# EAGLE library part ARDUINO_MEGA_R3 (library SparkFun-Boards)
Arduino Mega R3 ATmega2560 R3 compatible footprint. SparkFun Products: Arduino Mega 2560 R3
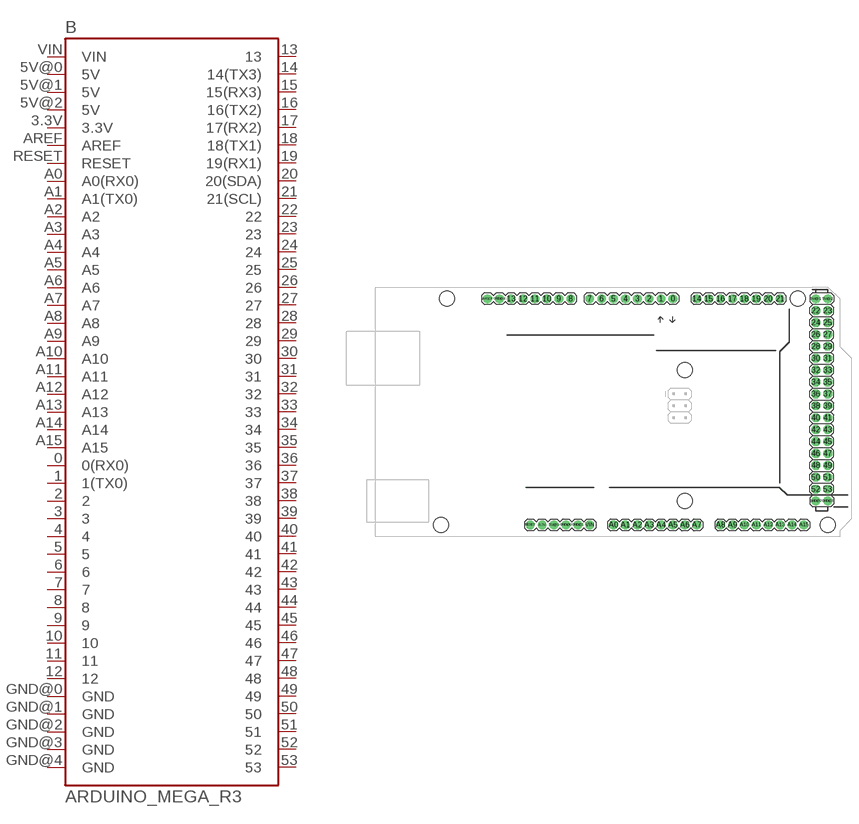
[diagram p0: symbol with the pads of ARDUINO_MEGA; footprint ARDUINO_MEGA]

Designator prefix B

## ARDUINO_MEGA_R3FULL  [ARDUINO_MEGA]
0  0(RX0)
1  1(TX0)
2  2
3  3
3.3V  3.3V
4  4
5  5
5V@0  5V
5V@1  5V
5V@2  5V
6  6
7  7
8  8
9  9
10  10
11  11
12  12
13  13
14  14(TX3)
15  15(RX3)
16  16(TX2)
17  17(RX2)
18  18(TX1)
19  19(RX1)
20  20(SDA)
21  21(SCL)
22  22
23  23
24  24
25  25
26  26
27  27
28  28
29  29
30  30
31  31
32  32
33  33
34  34
35  35
36  36
37  37
38  38
39  39
40  40
41  41
42  42
43  43
44  44
45  45
46  46
47  47
48  48
49  49
50  50
51  51
52  52
53  53
A0  A0(RX0)
A1  A1(TX0)
A2  A2
A3  A3
A4  A4
A5  A5
A6  A6
A7  A7
A8  A8
A9  A9
A10  A10
A11  A11
A12  A12
A13  A13
A14  A14
A15  A15
AREF  AREF
GND@0  GND
GND@1  GND
GND@2  GND
GND@3  GND
GND@4  GND
RESET  RESET
VIN  VIN

## Footprint ARDUINO_MEGA (pad centres in mm)
Arduino MEGA R3 footprint Specifications: Pin count:82 Area:4x2.15 in Example device(s): Arduino Mega R3
drill 1.016 pad 1.88: 0 13.97,24.13; 1 11.43,24.13; 2 8.89,24.13; 3 6.35,24.13; 3.3V -13.97,-24.13; 4 3.81,24.13; 5 1.27,24.13; 5V@0 -11.43,-24.13; 5V@1 44.45,24.13; 5V@2 46.99,24.13; 6 -1.27,24.13; 7 -3.81,24.13; 8 -7.874,24.13; 9 -10.414,24.13; 10 -12.954,24.13; 11 -15.494,24.13; 12 -18.034,24.13; 13 -20.574,24.13; 14 19.05,24.13; 15 21.59,24.13; 16 24.13,24.13; 17 26.67,24.13; 18 29.21,24.13; 19 31.75,24.13; 20 34.29,24.13; 21 36.83,24.13; A0 1.27,-24.13; A1 3.81,-24.13; A2 6.35,-24.13; A3 8.89,-24.13; A4 11.43,-24.13; A5 13.97,-24.13; A6 16.51,-24.13; A7 19.05,-24.13; A8 24.13,-24.13; A9 26.67,-24.13; A10 29.21,-24.13; A11 31.75,-24.13; A12 34.29,-24.13; A13 36.83,-24.13; A14 39.37,-24.13; A15 41.91,-24.13; AREF -25.654,24.13; GND@0 -8.89,-24.13; GND@1 -6.35,-24.13; GND@2 44.45,-19.05; GND@3 46.99,-19.05; GND@4 -23.114,24.13; RESET -16.51,-24.13; VIN -3.81,-24.13
drill 1.016 pad 1.88 octagon: 22 44.45,21.59; 23 46.99,21.59; 24 44.45,19.05; 25 46.99,19.05; 26 44.45,16.51; 27 46.99,16.51; 28 44.45,13.97; 29 46.99,13.97; 30 44.45,11.43; 31 46.99,11.43; 32 44.45,8.89; 33 46.99,8.89; 34 44.45,6.35; 35 46.99,6.35; 36 44.45,3.81; 37 46.99,3.81; 38 44.45,1.27; 39 46.99,1.27; 40 44.45,-1.27; 41 46.99,-1.27; 42 44.45,-3.81; 43 46.99,-3.81; 44 44.45,-6.35; 45 46.99,-6.35; 46 44.45,-8.89; 47 46.99,-8.89; 48 44.45,-11.43; 49 46.99,-11.43; 50 44.45,-13.97; 51 46.99,-13.97; 52 44.45,-16.51; 53 46.99,-16.51
hole 3.2 at -34.29,24.13
hole 3.2 at -35.56,-24.13
hole 3.2 at 16.51,8.89
hole 3.2 at 16.51,-19.05
hole 3.2 at 40.64,24.13
hole 3.2 at 46.99,-24.13

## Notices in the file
Licensing: Creative Commons ShareAlike 4.0 International - https://creativecommons.org/licenses/by-sa/4.0
